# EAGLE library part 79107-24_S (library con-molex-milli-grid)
RECEPTACAL
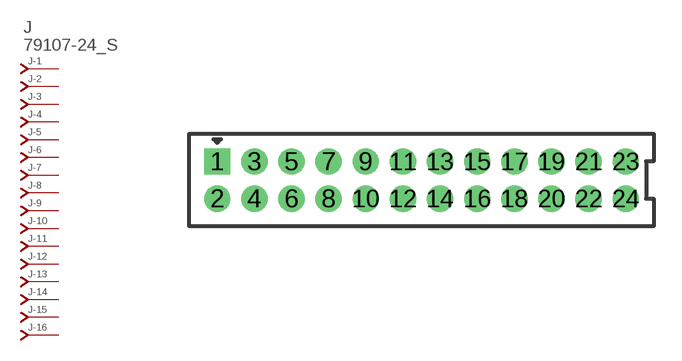
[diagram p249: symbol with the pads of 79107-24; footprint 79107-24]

Designator prefix J; gates -1=J-NV -2=J-N -3=J-N -4=J-N -5=J-N -6=J-N -7=J-N -8=J-N -9=J-N -10=J-N -11=J-N -12=J-N -13=J-N -14=J-N -15=J-N -16=J-N -17=J-N -18=J-N -19=J-N -20=J-N -21=J-N -22=J-N -23=J-N -24=J-N

## 79107-24_S  [79107-24]
1  -1:J  pas
2  -2:J  pas
3  -3:J  pas
4  -4:J  pas
5  -5:J  pas
6  -6:J  pas
7  -7:J  pas
8  -8:J  pas
9  -9:J  pas
10  -10:J  pas
11  -11:J  pas
12  -12:J  pas
13  -13:J  pas
14  -14:J  pas
15  -15:J  pas
16  -16:J  pas
17  -17:J  pas
18  -18:J  pas
19  -19:J  pas
20  -20:J  pas
21  -21:J  pas
22  -22:J  pas
23  -23:J  pas
24  -24:J  pas

## Footprint 79107-24 (pad centres in mm)
RECEPTACAL Dual Row, Vertical, Through-Hole
drill 0.914 square: 1 -11,1
drill 0.914: 2 -11,-1; 3 -9,1; 4 -9,-1; 5 -7,1; 6 -7,-1; 7 -5,1; 8 -5,-1; 9 -3,1; 10 -3,-1; 11 -1,1; 12 -1,-1; 13 1,1; 14 1,-1; 15 3,1; 16 3,-1; 17 5,1; 18 5,-1; 19 7,1; 20 7,-1; 21 9,1; 22 9,-1; 23 11,1; 24 11,-1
